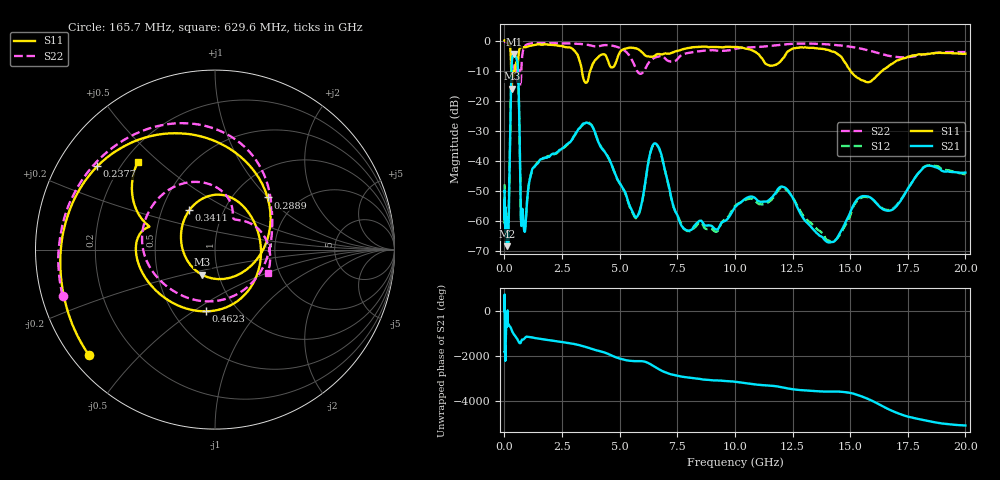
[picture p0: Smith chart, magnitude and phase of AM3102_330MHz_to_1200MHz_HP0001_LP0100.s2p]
! Date/Time: Tue, Sep 11, 2018 5:09 PM
! Network Analyzer: Agilent Technologies E8362B Rev: A.07.50.63
! Sweep from 0.010 to 20.000 GHz, 1601 Points, Sweep Type: LOG
! Power Supply: 4.950 V, 0.001 A
# Hz S DB R 50
!freq MagS11 AngS11 MagS21 AngS21 MagS12 AngS12 MagS22 AngS22
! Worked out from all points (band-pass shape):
!   1601 points, 10 MHz to 20 GHz, reference 50 ohm
!   highest |S21| = -4.43 dB at 412.5 MHz (marker M1); lowest = -68.3 dB at 113.3 MHz (marker M2)
!   |S21| within 3 dB of the highest: 320.7 MHz to 569 MHz (248.3 MHz wide, 55.8 % of centre)
!   lowest |S11| = -16.0 dB at 316.2 MHz (marker M3), VSWR 1.37, Z = 41.8 - j12 ohm
!   |S11| at or under -10 dB: 295.5 MHz to 444.8 MHz (149.3 MHz wide, 40.3 % of centre); 3.362 GHz to 3.726 GHz (364.1 MHz wide, 10.3 % of centre); 15.01 GHz to 16.4 GHz (1.392 GHz wide, 8.87 % of centre)
!   |S22| runs from -15.2 to -0.2 dB; largest |S21 - S12| = 0.0097
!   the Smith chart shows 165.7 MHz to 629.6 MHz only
!   S11 on the Smith chart (normalised r, x): 165.7 MHz: 0.05, -0.36; 237.7 MHz: 0.12, +0.31; 288.9 MHz: 1.42, +0.99; 341.1 MHz: 0.69, +0.32; 462.3 MHz: 0.72, -0.56; 629.6 MHz: 0.25, +0.43
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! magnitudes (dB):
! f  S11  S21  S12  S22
! 10 MHz  0.0  -50.1  -47.8  -0.2
! 35.55 MHz  0.0  -60.6  -62.7  -0.4
! 113.3 MHz  -0.4  -68.3  -62.1  -0.7
! 126.4 MHz  -0.4  -62.6  -63.2  -0.8
! 165.7 MHz  -0.8  -66.2  -65.2  -1.0
! 237.7 MHz  -1.9  -37.2  -37.3  -1.8
! 288.9 MHz  -7.7  -15.1  -15.2  -4.0
! 316.2 MHz  -16.0  -8.1  -8.1  -7.7
! 341.1 MHz  -11.6  -5.8  -5.9  -10.4
! 412.5 MHz  -11.8  -4.4  -4.5  -9.4
! 447.2 MHz  -9.9  -4.7  -4.7  -7.9
! 462.3 MHz  -9.2  -4.9  -4.9  -7.6
! 629.6 MHz  -3.7  -19.6  -19.6  -9.9
! 733 MHz  -2.2  -61.4  -60.7  -10.3
! 1.59 GHz  -1.4  -39.4  -39.5  -0.9
! 3.668 GHz  -11.6  -27.6  -27.3  -1.5
! 5.652 GHz  -2.5  -58.3  -58.7  -8.5
! 6.549 GHz  -4.9  -34.2  -34.4  -5.6
! 7.958 GHz  -2.5  -63.2  -63.3  -4.2
! 12.03 GHz  -6.4  -48.5  -48.9  -1.4
! 14.07 GHz  -3.2  -67.1  -66.5  -1.3
! 20 GHz  -4.4  -43.9  -44.4  -3.8
